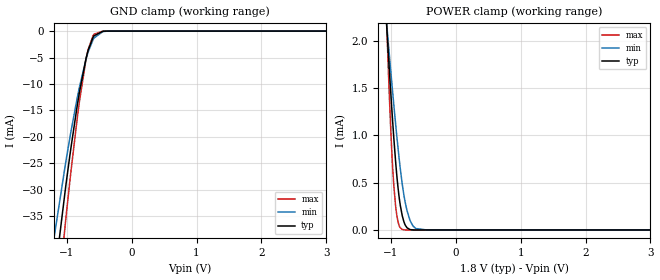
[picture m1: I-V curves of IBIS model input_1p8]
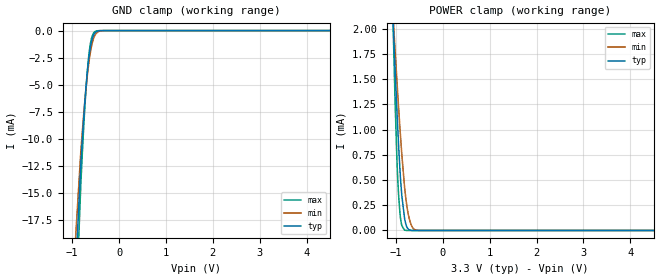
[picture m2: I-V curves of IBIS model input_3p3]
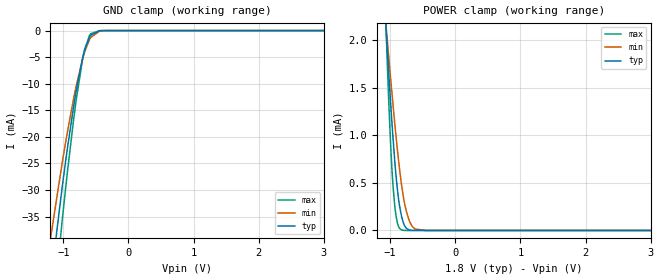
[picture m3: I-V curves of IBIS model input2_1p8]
|Texas Instruments Incorporated
| DIX4192 Integrated Digital Audio Interface Receiver and Transmitter
| Marketing part#   Digital Voltage Range   Package-type   #pins
| DIX4192   1.65V-3.6V   TQFP   48
[IBIS Ver]   4.1
[File name]   dix4192.ibs
[Date]   04/24/2017
[File Rev]   1.0
[Source]
| Texas Instruments Incorporated.
| Analog-eLab Design Center, HPA
| 12500 TI Blvd
| Dallas, TX -75243
[Notes]   Revision History:
| Rev 1.0: 04/24/2017
| - Initial version of the model
| - Model generated from simulations in SPECTRE
| - Model matched to SPICE simulation
| - C_comp although listed in numerical order of value are
|   obtained from varying PVT conditions. For PVT conditions for
|   each specific value refer the buffer description under
|   respective [Model]. IBIS model user is responsible for using
|   appropriate C_comp to simulate for Signal Integrity.
[Disclaimer]
| This model is designed as an aid for customers of Texas Instruments.
| TI and its licensors and suppliers make no warranties, either expressed
| or implied, with respect to this  model, including the warranties of
| merchantability or fitness for a particular purpose. The model is
| provided solely on an "as is" basis. The entire risk as to its quality
| and performance is with the customer.
[Copyright]
(C) Copyright 2017 Texas Instruments Incorporated.All rights reserved.
|   DIX4192
[Component]   DIX4192
[Manufacturer]  TI
[Package]   |48 TQFP
|   typ   min   max
R_pkg   0   0   0
L_pkg   0   0   0
C_pkg   0   0   0
|   l
[Pin]  signal_name model_name   R_pin   L_pin   C_pin
1   RX1+   nc   NA   NA   NA
2   RX1-   nc   NA   NA   NA
3   RX2+   nc   NA   NA   NA
4   RX2-   nc   NA   NA   NA
5   RX3+   nc   NA   NA   NA
6   RX3-   nc   NA   NA   NA
7   RX4+   nc   NA   NA   NA
8   RX4-   nc   NA   NA   NA
9   VCC   power   NA   NA   NA
10   AGND   gnd   NA   NA   NA
11   LOCK   output1   NA   NA   NA
12   RXCKO   output1   NA   NA   NA
13   RXCKI   input   NA   NA   NA
14   NC   nc   NA   NA   NA
15   NC   nc   NA   NA   NA
16   DGND1   gnd   NA   NA   NA
17   VDD18   power   NA   NA   NA
18   CPM   input   NA   NA   NA
19   _CS/A0   input   NA   NA   NA
20   CCLK/SCL   input   NA   NA   NA
21   CDIN/A1   input   NA   NA   NA
22   CDOUT/SDA   io   NA   NA   NA
23   _INT   int   NA   NA   NA
24   _RST   input   NA   NA   NA
25   MCLK   input   NA   NA   NA
26   GPO1   output1   NA   NA   NA
27   GPO2   output1   NA   NA   NA
28   GPO3   output1   NA   NA   NA
29   GPO4   output1   NA   NA   NA
30   DGND2   gnd   NA   NA   NA
31   TX-   nc   NA   NA   NA
32   TX+   nc   NA   NA   NA
33   VDD33   power   NA   NA   NA
34   AESOUT   output1   NA   NA   NA
35   BLS   io1   NA   NA   NA
36   SYNC   output1   NA   NA   NA
37   BCKA   io2   NA   NA   NA
38   LRCKA   io2   NA   NA   NA
39   SDINA   input2   NA   NA   NA
40   SDOUTA   output1   NA   NA   NA
41   NC   nc   NA   NA   NA
42   VIO   power   NA   NA   NA
43   DGND3   gnd   NA   NA   NA
44   BGND   gnd   NA   NA   NA
45   SDOUTB   output1   NA   NA   NA
46   SDINB   input2   NA   NA   NA
47   LRCKB   io2   NA   NA   NA
48   BCKB   io2   NA   NA   NA
|   Model Selectors
[Model Selector] input
input_1p8   1.8V  digital Input
input_3p3   3.3V  digital Input
[Model Selector] input2
input2_1p8   1.8V  digital Input
input2_3p3   3.3V  digital Input
[Model Selector] output1
output1_1p8   1.8V  digital Output
output1_3p3   3.3V  digital Output
[Model Selector] io
io_1p8   1.8V  digital Output
io_3p3   3.3V  digital Output
sda_1p8   1.8V  digital I/O_open_drain
sda_3p3   3.3V  digital I/O_open_drain
[Model Selector] io1
io1_1p8   1.8V  digital I/O
io1_3p3   3.3V  digital I/O
[Model Selector] io2
io2_1p8   1.8V  digital I/O
io2_3p3   3.3V  digital I/O
[Model Selector] int
int_1p8   1.8V  digital I/O_open_drain
int_3p3   3.3V  digital I/O_open_drain
| Models and submodels in the file (16): input_1p8 (Input), input_3p3 (Input), input2_1p8 (Input), input2_3p3 (Input), output1_1p8 (3-state), output1_3p3 (3-state), io_1p8 (3-state), io_3p3 (3-state), sda_1p8 (I/O_open_drain), sda_3p3 (I/O_open_drain), io1_1p8 (I/O), io1_3p3 (I/O), io2_1p8 (I/O), io2_3p3 (I/O), int_1p8 (I/O_open_drain), int_3p3 (I/O_open_drain)
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|   input_1p8 Model
[Model]   input_1p8
Model_type   Input
Vinl = 0.54
Vinh = 1.26
|   typ   min   max
C_comp   30.3138pF   24.4141pF   36.1111pF
[Model spec]
|subparameter
Vinl   0.54   0.495   0.585
Vinh   1.26   1.155   1.365
| Where Nom  PVT is Nominal Process, 1.8V, 27C
|   Fast PVT is Strong Process,  1.95V, -40C
|   Slow PVT is Weak Process,   1.65V, 105C
[Voltage Range]   1.8   1.65   1.95
[Temperature Range]   27   105   -40
[Power Clamp Reference]   1.8   1.65   1.95
[GND Clamp Reference]   0   0   0
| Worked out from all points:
|   GND clamp passes 1 mA (typ) near -0.59 V on its own axis
|   POWER clamp passes 1 mA (typ) near -0.96 V on its own axis
[GND Clamp]
|   Voltage   I(typ)   I(min)   I(max)
-1.8V     -121.1mA   -94.72mA   -158.6mA
-1.233V   -51.05mA   -42mA      -62.41mA
-1.017V   -29.41mA   -24.84mA   -35.72mA
-936mV    -22.06mA   -19mA      -26.53mA
-806.4mV  -11.65mA   -10.66mA   -13.42mA
-703.8mV  -5.197mA   -5.331mA   -5.369mA
-682.2mV  -4.132mA   -4.411mA   -4.087mA
-595.8mV  -1.194mA   -1.647mA   -871.2uA
-579.6mV  -883uA     -1.305mA   -595uA
-444.6mV  -34uA      -103.4uA   -9.415uA
-352.8mV  -1.917uA   -11.95uA   -99.03nA
3.6V      0A         0A         0A
[POWER Clamp]
|   Voltage   I(typ)   I(min)   I(max)
-1.8V     11.51mA    8.536mA    18.67mA
-1.076V   2.271mA    2.258mA    2.367mA
-1.039V   1.838mA    1.954mA    1.652mA
-995.4mV  1.365mA    1.616mA    939.7uA
-957.6mV  983.6uA    1.33mA     479.5uA
-903.6mV  528.3uA    946.2uA    129.2uA
-865.8mV  303.5uA    703.7uA    34.04uA
-828mV    156.5uA    493.5uA    6.61uA
-752.4mV  22.76uA    203uA      76.23nA
-698.4mV  3.563uA    88.91uA    0A
-617.4mV  41.9nA     14.98uA    0A
3.6V      0A         0A         0A
|   input_3p3 Model
[Model]   input_3p3
Model_type   Input
Vinl = 0.99
Vinh = 2.31
|   typ   min   max
C_comp   30.3138pF   24.4141pF   36.1111pF
[Model spec]
|subparameter
Vinl   0.99   0.90   1.08
Vinh   2.31   2.10   2.52
| Where nom  PVT is Nominal Process, 3.3V, 27C
|   Fast PVT is Strong Process,  3.6V, -40C
|   Slow PVT is Weak Process,   3.0V, 105C
[Voltage Range]   3.3   3   3.6
[Temperature Range]   27   105   -40
[Power Clamp Reference]   3.3   3   3.6
[GND Clamp Reference]   0   0   0
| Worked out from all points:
|   GND clamp passes 1 mA (typ) near -0.59 V on its own axis
|   POWER clamp passes 1 mA (typ) near -0.96 V on its own axis
[GND Clamp]
|   Voltage   I(typ)   I(min)   I(max)
-3.3V     -1.038A    -961.1mA   -1.11A
-1.142V   -41.61mA   -34.51mA   -50.84mA
-815.1mV  -12.28mA   -11.17mA   -14.21mA
-765.6mV  -8.842mA   -8.374mA   -9.888mA
-726mV    -6.411mA   -6.358mA   -6.858mA
-686.4mV  -4.33mA    -4.583mA   -4.322mA
-656.7mV  -3.038mA   -3.436mA   -2.811mA
-627mV    -2.016mA   -2.465mA   -1.672mA
-587.4mV  -1.024mA   -1.463mA   -717.3uA
-498.3mV  -142.1uA   -316.3uA   -60.16uA
-260.7mV  0A         -705.9nA   0A
6.6V      0A         0A         0A
[POWER Clamp]
|   Voltage   I(typ)   I(min)   I(max)
-3.3V     31.5mA     22.11mA    54.06mA
-1.063V   2.111mA    2.146mA    2.099mA
-1.053V   1.997mA    2.066mA    1.911mA
-1.013V   1.555mA    1.753mA    1.213mA
-983.4mV  1.24mA     1.524mA    773.4uA
-943.8mV  854.9uA    1.228mA    359.1uA
-894.3mV  464.9uA    884uA      96.47uA
-815.1mV  120.1uA    431uA      3.519uA
-755.7mV  25.1uA     212uA      70.96nA
-696.3mV  3.16uA     85.49uA    0A
-547.8mV  0A         1.94uA     0A
6.6V      0A         0A         0A
|   input2_1p8 Model
[Model]   input2_1p8
Model_type   Input
Vinl = 0.54
Vinh = 1.26
|   typ   min   max
C_comp   30.3138pF   24.5267pF   36.1111pF
[Model spec]
|subparameter
Vinl   0.54   0.495   0.585
Vinh   1.26   1.155   1.365
| Where nom  PVT is Nominal Process, 1.8V, 27C
|   Fast PVT is Strong Process,  1.95V, -40C
|   Slow PVT is Weak Process,   1.65V, 105C
[Voltage Range]   1.8   1.65   1.95
[Temperature Range]   27   105   -40
[Power Clamp Reference]   1.8   1.65   1.95
[GND Clamp Reference]   0   0   0
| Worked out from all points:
|   GND clamp passes 1 mA (typ) near -0.59 V on its own axis
|   POWER clamp passes 1 mA (typ) near -0.96 V on its own axis
[GND Clamp]
|   Voltage   I(typ)   I(min)   I(max)
-1.8V     -121.2mA   -94.82mA   -158.7mA
-1.233V   -51.1mA    -42.05mA   -62.47mA
-1.017V   -29.44mA   -24.88mA   -35.74mA
-936mV    -22.08mA   -19.03mA   -26.54mA
-806.4mV  -11.66mA   -10.68mA   -13.42mA
-703.8mV  -5.199mA   -5.343mA   -5.369mA
-682.2mV  -4.134mA   -4.421mA   -4.087mA
-595.8mV  -1.194mA   -1.652mA   -871.2uA
-579.6mV  -883.1uA   -1.308mA   -595uA
-444.6mV  -34.01uA   -103.6uA   -9.417uA
-352.8mV  -1.917uA   -11.97uA   -98.92nA
3.6V      0A         0A         0A
[POWER Clamp]
|   Voltage   I(typ)   I(min)   I(max)
-1.8V     11.51mA    8.536mA    18.67mA
-1.076V   2.271mA    2.258mA    2.367mA
-1.039V   1.838mA    1.954mA    1.652mA
-995.4mV  1.365mA    1.616mA    939.7uA
-957.6mV  983.6uA    1.33mA     479.5uA
-903.6mV  528.3uA    946.2uA    129.2uA
-865.8mV  303.5uA    703.7uA    34.04uA
-828mV    156.5uA    493.5uA    6.61uA
-752.4mV  22.76uA    203uA      76.16nA
-698.4mV  3.562uA    88.91uA    0A
-617.4mV  41.82nA    14.98uA    0A
3.6V      0A         0A         0A
